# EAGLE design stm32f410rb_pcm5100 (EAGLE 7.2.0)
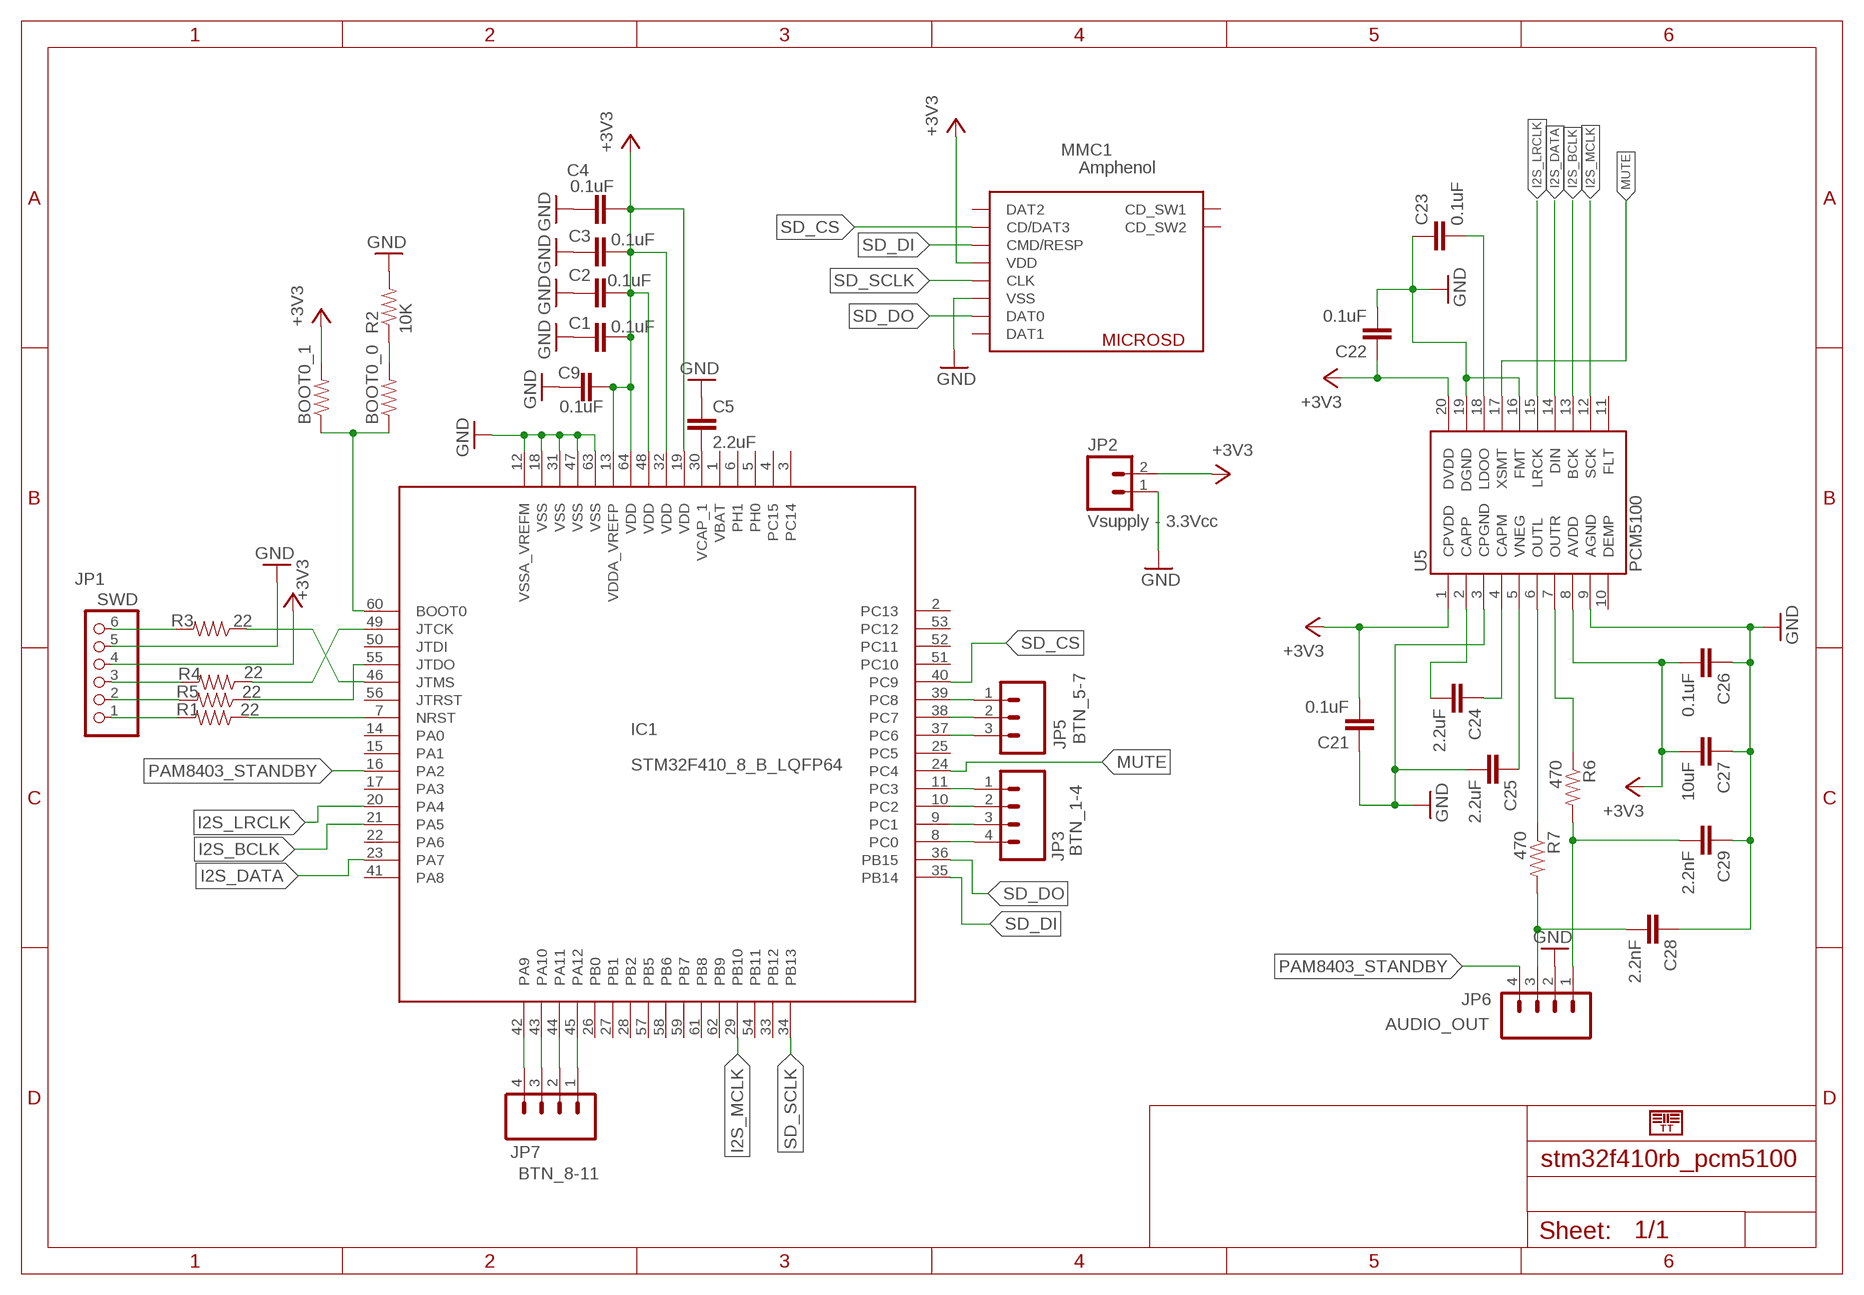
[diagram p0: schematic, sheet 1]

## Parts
BOOT0_0  RESISTOR0603-RES  [0603-RES]
BOOT0_1  RESISTOR0603-RES  [0603-RES]
C1  0.1uF  CAP0805  [0805]
C2  0.1uF  CAP0805  [0805]
C3  0.1uF  CAP0805  [0805]
C4  0.1uF  CAP0805  [0805]
C5  2.2uF  CAP0805  [0805]
C9  0.1uF  CAP0805  [0805]
C21  0.1uF  CAP0805  [0805]
C22  0.1uF  CAP0805  [0805]
C23  0.1uF  CAP0805  [0805]
C24  2.2uF  CAP0805  [0805]
C25  2.2uF  CAP0805  [0805]
C26  0.1uF  CAP0805  [0805]
C27  10uF  CAP0805  [0805]
C28  2.2nF  CAP0805  [0805]
C29  2.2nF  CAP0805  [0805]
IC1  STM32F410_8_B_LQFP64  [LQFP64]
JP1  SWD  PINHD-1X6  [1X06]
JP2  Vsupply - 3.3Vcc  M023.5MM  [SCREWTERMINAL-3.5MM-2]
JP3  BTN_1-4  M04SCREW  [SCREWTERMINAL-3.5MM-4]
JP5  BTN_5-7  M03SCREW  [SCREWTERMINAL-3.5MM-3]
JP6  AUDIO_OUT  M04SCREW  [SCREWTERMINAL-3.5MM-4]
JP7  BTN_8-11  M04SCREW  [SCREWTERMINAL-3.5MM-4]
MMC1  Amphenol  MICROSD_AMPHENOL  [MICROSD_AMPHENOL]
R1  22  RESISTOR0805-RES  [0805]
R2  10K  RESISTOR0805-RES  [0805]
R3  22  RESISTOR0805-RES  [0805]
R4  22  RESISTOR0805-RES  [0805]
R5  22  RESISTOR0805-RES  [0805]
R6  470  RESISTOR0805-RES  [0805]
R7  470  RESISTOR0805-RES  [0805]
U5  PCM5100  [PW_R-PDSO-G20]

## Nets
GND: C1.2 C2.2 C3.2 C4.2 C5.1 C9.2 C21.1 C22.2 C23.1 C25.2 C26.1 C27.1 C28.1 C29.1 IC1.12(VSSA_VREFM) IC1.18(VSS) IC1.31(VSS) IC1.47(VSS) IC1.63(VSS) JP1.5 JP2.1 JP6.2 MMC1.VSS R2.2 U5.3(CPGND) U5.9(AGND) U5.16(FMT) U5.19(DGND)
I2S_BCLK: IC1.21(PA5) U5.13(BCK)
I2S_DATA: IC1.23(PA7) U5.14(DIN)
I2S_LRCLK: IC1.20(PA4) U5.15(LRCK)
I2S_MCLK: IC1.29(PB10) U5.12(SCK)
LOUTL: C28.2 JP6.3 R7.2
LOUTR: C29.2 JP6.1 R6.2
MUTE: IC1.24(PC4) U5.17(XSMT)
N$1: IC1.11(PC3) JP3.1
N$2: IC1.10(PC2) JP3.2
N$3: IC1.9(PC1) JP3.3
N$4: IC1.8(PC0) JP3.4
N$5: C5.2 IC1.30(VCAP_1)
N$6: IC1.7(NRST) R1.1
N$7: IC1.49(JTCK) R4.1
N$8: IC1.55(JTDO) R5.1
N$9: IC1.46(JTMS) R3.1
N$10: BOOT0_0.2 R2.1
N$12: IC1.39(PC8) JP5.1
N$13: IC1.38(PC7) JP5.2
N$14: C23.2 U5.18(LDOO)
N$15: R6.1 U5.7(OUTR)
N$16: C24.2 U5.2(CAPP)
N$17: C24.1 U5.4(CAPM)
N$18: C25.1 U5.5(VNEG)
N$19: R7.1 U5.6(OUTL)
N$20: BOOT0_0.1 BOOT0_1.1 IC1.60(BOOT0)
N$21: IC1.37(PC6) JP5.3
N$22: IC1.45(PA12) JP7.1
N$23: IC1.44(PA11) JP7.2
N$24: IC1.43(PA10) JP7.3
N$25: IC1.42(PA9) JP7.4
N$26: JP1.6 R3.2
N$27: JP1.3 R4.2
N$28: JP1.2 R5.2
N$29: JP1.1 R1.2
PAM8403_STANDBY: IC1.16(PA2) JP6.4
SD_CS: IC1.40(PC9) MMC1.CD/DAT3
SD_DI: IC1.35(PB14) MMC1.CMD/RESP
SD_DO: IC1.36(PB15) MMC1.DAT0
SD_SCLK: IC1.34(PB13) MMC1.CLK
VCC: BOOT0_1.2 C1.1 C2.1 C3.1 C4.1 C9.1 C21.2 C22.1 C26.2 C27.2 IC1.13(VDDA_VREFP) IC1.19(VDD) IC1.32(VDD) IC1.48(VDD) IC1.64(VDD) JP1.4 JP2.2 MMC1.VDD U5.1(CPVDD) U5.8(AVDD) U5.20(DVDD) ; supply symbol labelled +3V3
Unconnected: IC1.1(VBAT) IC1.2(PC13) IC1.3(PC14) IC1.4(PC15) IC1.5(PH0) IC1.6(PH1) IC1.14(PA0) IC1.15(PA1) IC1.17(PA3) IC1.22(PA6) IC1.25(PC5) IC1.26(PB0) IC1.27(PB1) IC1.28(PB2) IC1.33(PB12) IC1.41(PA8) IC1.50(JTDI) IC1.51(PC10) IC1.52(PC11) IC1.53(PC12) IC1.54(PB11) IC1.56(JTRST) IC1.57(PB5) IC1.58(PB6) IC1.59(PB7) IC1.61(PB8) IC1.62(PB9) MMC1.CD_SW1 MMC1.CD_SW2 MMC1.DAT1 MMC1.DAT2 U5.10(DEMP) U5.11(FLT)

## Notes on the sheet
- TT

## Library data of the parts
BOOT0_0 BOOT0_1 R1-R7 = SparkFun-Passives:RESISTOR: Resistor
C1-C5 C9 C21-C29 = SparkFun-Passives:CAP: Capacitor
IC1 = pel_stm32:STM32F410_8_B_LQFP64: STM32F410_8_B_LQFP64.bsd edit this description Auto generated by make-symbol-device-package-bsdl.ulp Rev. 18 Source: STM32F410_8_B_LQFP64.bsd
JP1 = pinhead:PINHD-1X6: PIN HEADER
JP2 = SparkFun-Connectors:M02: Standard 2-pin 0.1" header. Use with; PROD_ID: CONN-08399
JP3 JP6 JP7 = SparkFun-Connectors:M04: Header 4 Standard 4-pin 0.1" header. Use with straight break away headers (SKU : PRT-00116), right angle break away headers (PRT-00553), swiss pins (PRT-00743), machine pins (PRT-00117), and female headers (PRT-00115). Molex polarized connector foot print use with SKU : PRT-08231 with associated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
JP5 = SparkFun-Connectors:M03: Header 3 Standard 3-pin 0.1" header. Use with straight break away headers (SKU : PRT-00116), right angle break away headers (PRT-00553), swiss pins (PRT-00743), machine pins (PRT-00117), and female headers (PRT-00115). Molex polarized connector foot print use with SKU : PRT-08232 with associated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
MMC1 = microsd_amphenol:MICROSD_AMPHENOL: AMPHENOL COMMERCIAL PRODUCTS The 114-00841-68 is a top mount microSD Memory Card Connector with gold-plated contact and tin-plated solder tail. http://ro.farnell.com/amphenol-commercial-products/114-00841-68/memory-card-connector-microsd/dp/2293708?CMP=i-ddd7-00001003
U5 = robertsonics:PCM5100: PCM5100 Stereo DAC

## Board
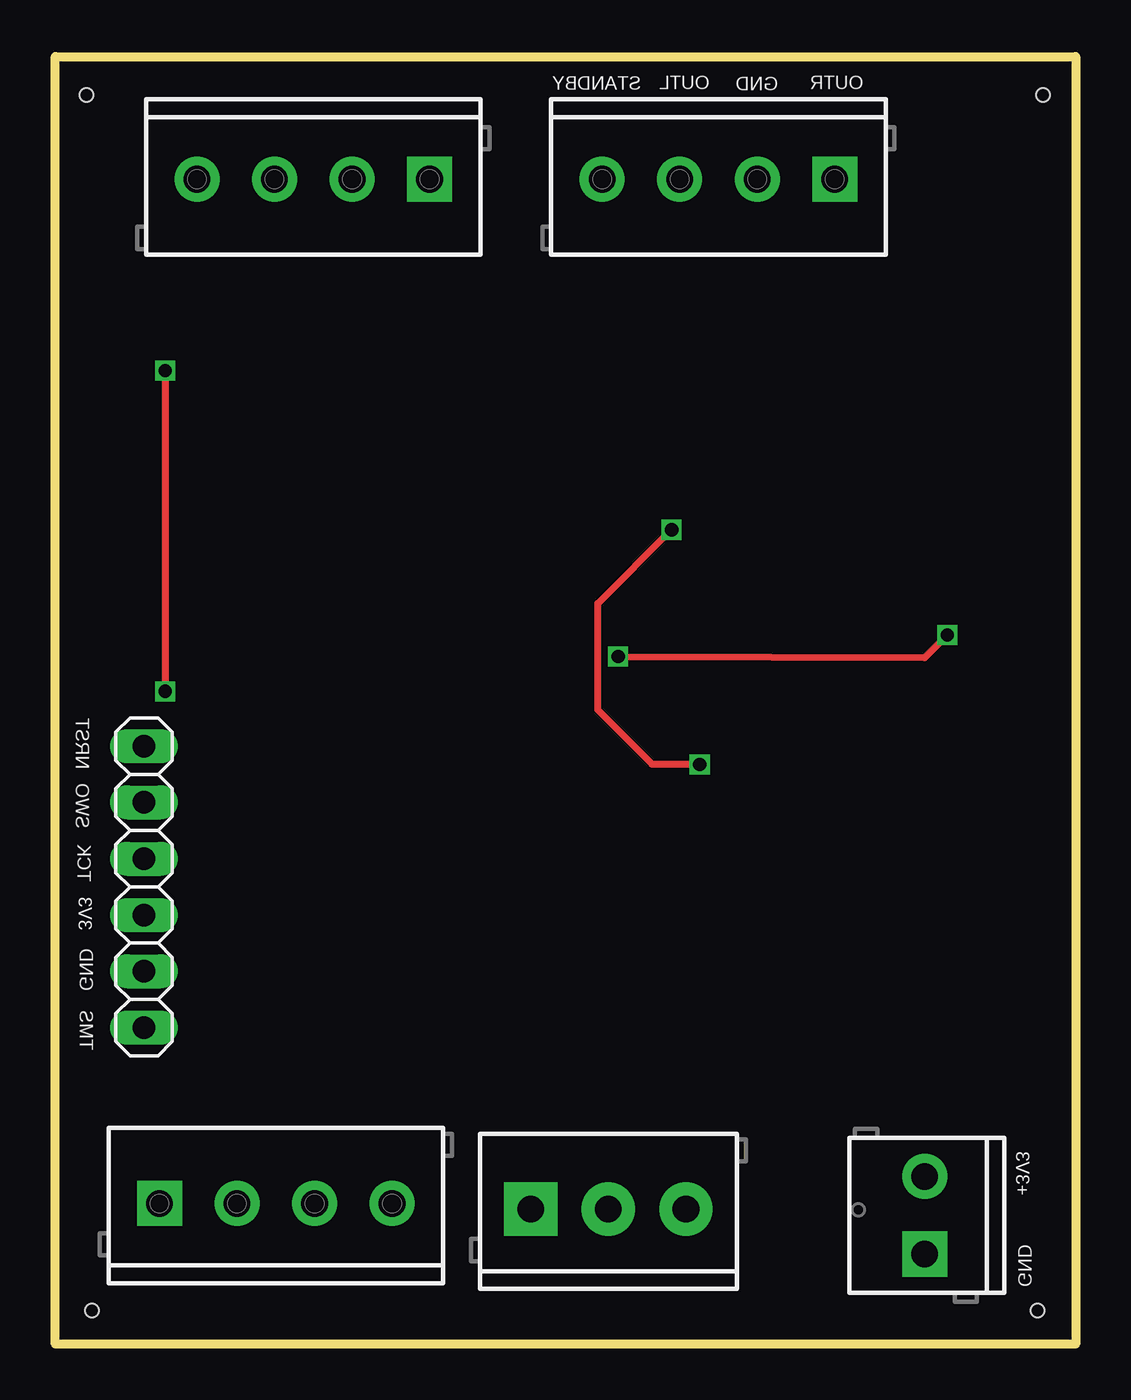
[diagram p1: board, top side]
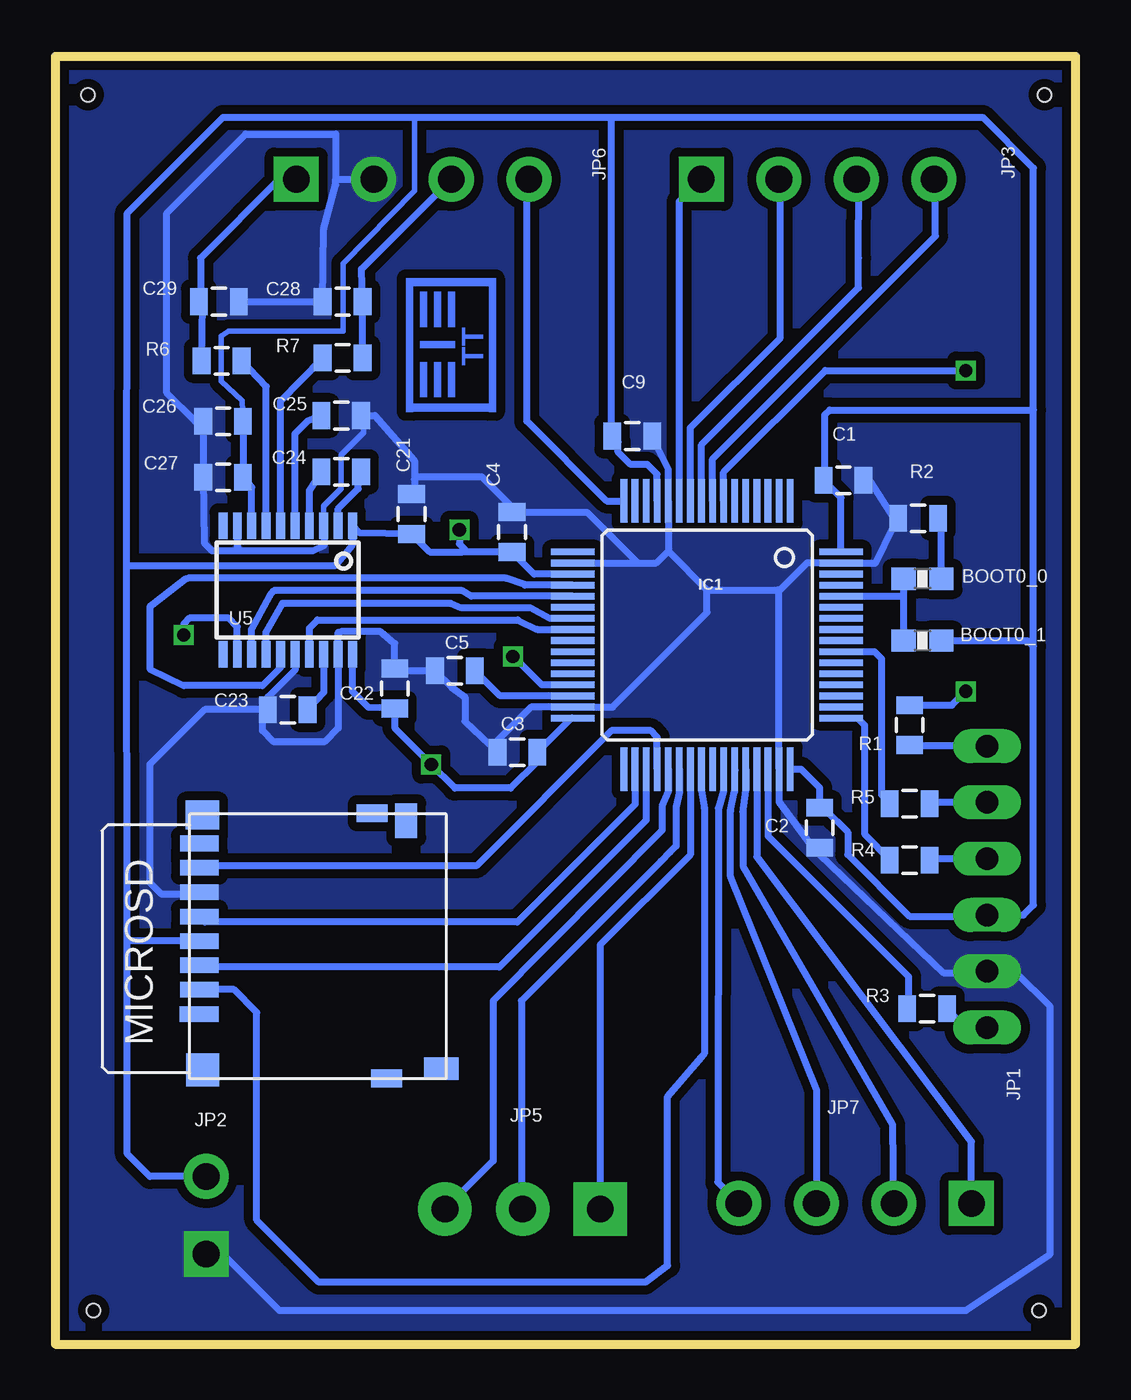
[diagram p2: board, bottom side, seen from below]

Size 46.05 x 58.17 mm. Coordinates in mm from the lower left corner, seen from the top.
Outline: 0,0 46.02,0 46.02,58.17 0,58.17
Outline: 0,58.09 0,0
Outline: 0,0 46.05,0 46.05,58.12 0,58.12 0,0
Copper layers (1*16): Top 0.035mm / dielectric 1.5mm / Bottom 0.035mm
Design rules "dirt_cheap_dirty_boards.v1 *": minimum track width 5mil, minimum drill 12mil, track to track 5mil, track to pad 5mil, pad to pad 5mil, via to via 5mil, smd to smd 0mil, copper to edge 10mil, drill to drill 10mil, minimum pad ring 10mil, minimum via ring 6mil, stop-mask expansion 2mil, vias tented up to drill 25mil, thermal gap 10mil
Holes 0.6 mm at 1.4,56.39 44.58,56.39 1.65,1.52 44.32,1.52

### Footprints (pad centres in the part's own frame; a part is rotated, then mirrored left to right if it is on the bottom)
0603-RES = smd 1.1 x 1: 1 -0.85,0; 2 0.85,0
0805 = smd 0.8 x 1.2: 1 -0.9,0; 2 0.9,0
LQFP64 = smd 1.962 x 0.3: 1 -6.05,3.75; 2 -6.05,3.25; 3 -6.05,2.75; 4 -6.05,2.25; 5 -6.05,1.75; 6 -6.05,1.25; 7 -6.05,0.75; 8 -6.05,0.25; 9 -6.05,-0.25; 10 -6.05,-0.75; 11 -6.05,-1.25; 12 -6.05,-1.75; 13 -6.05,-2.25; 14 -6.05,-2.75; 15 -6.05,-3.25; 16 -6.05,-3.75; 33 6.05,-3.75; 34 6.05,-3.25; 35 6.05,-2.75; 36 6.05,-2.25; 37 6.05,-1.75; 38 6.05,-1.25; 39 6.05,-0.75; 40 6.05,-0.25; 41 6.05,0.25; 42 6.05,0.75; 43 6.05,1.25; 44 6.05,1.75; 45 6.05,2.25; 46 6.05,2.75; 47 6.05,3.25; 48 6.05,3.75 | smd 0.3 x 1.962: 17 -3.75,-6.05; 18 -3.25,-6.05; 19 -2.75,-6.05; 20 -2.25,-6.05; 21 -1.75,-6.05; 22 -1.25,-6.05; 23 -0.75,-6.05; 24 -0.25,-6.05; 25 0.25,-6.05; 26 0.75,-6.05; 27 1.25,-6.05; 28 1.75,-6.05; 29 2.25,-6.05; 30 2.75,-6.05; 31 3.25,-6.05; 32 3.75,-6.05; 49 3.75,6.05; 50 3.25,6.05; 51 2.75,6.05; 52 2.25,6.05; 53 1.75,6.05; 54 1.25,6.05; 55 0.75,6.05; 56 0.25,6.05; 57 -0.25,6.05; 58 -0.75,6.05; 59 -1.25,6.05; 60 -1.75,6.05; 61 -2.25,6.05; 62 -2.75,6.05; 63 -3.25,6.05; 64 -3.75,6.05
1X06 = drill 1.016 long: 1 -6.35,0; 2 -3.81,0; 3 -1.27,0; 4 1.27,0; 5 3.81,0; 6 6.35,0
SCREWTERMINAL-3.5MM-2 = drill 1.2 pad 2.032 square: 1 0,0 | drill 1.2 pad 2.032: 2 3.5,0
SCREWTERMINAL-3.5MM-4 = drill 1.2 pad 2.032 square: 1 0,0 | drill 1.2 pad 2.032: 2 3.5,0; 3 7,0; 4 10.5,0
SCREWTERMINAL-3.5MM-3 = drill 1.2 pad 2.413 square: 1 0,0 | drill 1.2 pad 2.413: 2 3.5,0; 3 7,0
MICROSD_AMPHENOL = smd 0.7 x 1.75: CD/DAT3 2.1,-5.51; CLK -1.2,-5.51; CMD/RESP 1,-5.51; DAT0 -3.4,-5.51; DAT1 -4.5,-5.51; DAT2 3.21,-5.52; VDD -0.1,-5.51; VSS -2.3,-5.51 | smd 1 x 1.55: CD_SW1 5.66,5.41 | smd 1.55 x 1: CD_SW2 -5.53,3.82 | smd 1.3 x 1.5: NC1 -5.78,-5.38 | smd 1.5 x 1.5: NC2 5.72,-5.37 | smd 0.8 x 1.4: NC3 -5.86,2.29; NC_4 6.1,2.93
PW_R-PDSO-G20 = smd 0.4 x 1.2: 1 -2.925,-2.9; 2 -2.275,-2.9; 3 -1.625,-2.9; 4 -0.975,-2.9; 5 -0.325,-2.9; 6 0.325,-2.9; 7 0.975,-2.9; 8 1.625,-2.9; 9 2.275,-2.9; 10 2.925,-2.9; 11 2.925,2.9; 12 2.275,2.9; 13 1.625,2.9; 14 0.975,2.9; 15 0.325,2.9; 16 -0.325,2.9; 17 -0.975,2.9; 18 -1.625,2.9; 19 -2.275,2.9; 20 -2.925,2.9

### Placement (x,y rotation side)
BOOT0_0  6.91,34.54 0 bottom
BOOT0_1  6.91,31.75 0 bottom
C1  10.48,38.99 0 bottom
C2  11.56,23.3 270 bottom
C3  25.2,26.72 180 bottom
C4  25.44,36.65 90 bottom
C5  28.02,30.39 0 bottom
C9  20.02,40.98 0 bottom
C21  29.97,37.47 270 bottom
C22  30.73,29.59 90 bottom
C23  35.56,28.64 0 bottom
C24  33.15,39.37 0 bottom
C25  33.15,41.91 0 bottom
C26  38.48,41.66 0 bottom
C27  38.48,39.12 0 bottom
C28  33.08,47.05 0 bottom
C29  38.67,47.05 180 bottom
IC1  16.64,32 270 bottom
JP1  4,20.64 270 top
JP2  39.24,4.06 90 top
JP3  16.89,52.58 180 top
JP5  21.46,6.1 0 top
JP6  35.18,52.58 180 top
JP7  4.7,6.35 0 top
MMC1  34.04,18.1 270 bottom
R1  7.49,27.94 270 bottom
R2  7.11,37.27 180 bottom
R3  6.71,15.14 0 bottom
R4  7.49,21.84 0 bottom
R5  7.49,24.38 0 bottom
R6  38.54,44.39 180 bottom
R7  33.08,44.51 0 bottom
U5  35.56,34.04 180 bottom

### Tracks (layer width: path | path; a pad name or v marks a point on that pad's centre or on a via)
GND
  Bottom 0.254: U5.3 33.93,37.82 33.15,38.61 33.15,40.13 32.13,41.15 32.13,41.49 C25.2
  Bottom 0.305: 13.39,33.98 IC1.47 13.39,25.55 13.39,24.46 11.86,22.4 C2.2 11.56,22.1 5.97,16.76 4.06,16.76 JP1.5 3.94,16.76 2.67,16.76 1.14,15.24 1.14,4.06 4.95,1.52 35.94,1.52 38.48,4.06 JP2.1 | 18.39,35.79 IC1.12 18.39,39.49 C9.2 | 18.39,35.79 16.64,34.04 | 16.64,34.04 13.44,34.04 13.39,33.98 | IC1.18 19.76,35.25 | 19.76,35.25 18.92,35.25 18.39,35.79 | 8,37.31 R2.2 | 8.23,37.31 8.23,36.88 9.02,35.25 IC1.63 12.12,35.25 13.39,33.98 | 8.23,37.31 8.05,37.27 R2.2 | C29.1 C28.1 33.93,50.32 33.4,52.32 33.4,52.58 | C25.2 31.62,41.91 29.85,39.88 29.85,39.04 | 29.85,39.04 29.85,38.44 C21.1 | U5.9 37.84,35.93 37.72,35.81 | 37.72,35.81 34.42,35.81 33.91,36.07 33.91,36.91 U5.3 | 37.72,35.81 38.99,35.81 39.33,36.16 C27.1 C26.1 39.75,41.66 41.02,42.93 41.02,51.05 37.46,54.61 33.4,54.61 33.4,52.58 | 33.4,52.58 JP6.2 | C23.1 39.31,28.64 41.78,26.16 41.78,20.83 41.27,20.32 39.62,20.32 MMC1.VSS | C22.2 30.73,31.62 31.37,32.16 33.15,32.16 33.28,32.12 U5.19 33.28,27.8 33.91,27.18 36.2,27.18 36.7,27.69 36.7,28.35 C23.1 | U5.16 35.23,30.42 36.45,29.21 36.45,28.68 C23.1 | 30.71,30.42 C22.2 | 16.64,34.04 16.64,33.02 20.9,28.75 IC1.31 24.59,28.75 26.09,27.25 26.09,26.73 C3.2 27.56,28.11 27.56,29.21 28.16,29.63 C5.1 30.63,30.39 C22.2 | C1.2 9.63,38.94 9.27,38.94 8.23,37.31 | 8.23,37.31 R2.2 | 29.85,39.04 29.74,39.14 26.8,39.14 25.44,37.78 C4.2 22.06,37.55 19.76,35.25
  pour Bottom (isolate 0.406, no thermals): -0.03,58.19 46.05,58.19 46.05,-0.08 -0.03,-0.08
I2S_BCLK
  Bottom 0.305: U5.13 37.21,31.16 37.21,32.26 36.37,33.78 36.19,34.01 27.69,34.01 27.28,33.75 IC1.21
I2S_DATA
  Bottom 0.305: U5.14 36.53,32.17 35.81,33.43 28.19,33.43 27.71,33.22 24.61,33.22 23.74,32.75 IC1.23
I2S_LRCLK
  Bottom 0.305: U5.15 35.88,30.54 36.7,29.72 40.26,29.72 41.78,30.48 41.78,33.27 40.17,34.53 40.07,34.57 25.73,34.57 24.88,34.28 24.86,34.25 IC1.20
I2S_MCLK  (via drill 0.6)
  Top 0.305: v25.4,31.04 39.24,30.99 v40.26,32
  Bottom 0.305: IC1.29 24.09,29.75 25.02,30.68 v25.4,31.04 | U5.12 37.84,32.37 38.23,32.77 40,32.77 40.26,32.51 v40.26,32
LOUTL
  Bottom 0.305: R7.2 C28.2 32.23,48.52 JP6.3
LOUTR
  Bottom 0.305: R6.2 39.39,46.93 C29.2 39.5,47.08 39.5,49.02 35.94,52.58 JP6.1
MUTE
  Bottom 0.305: IC1.24 22.39,32.26 24.31,32.26 25.15,32.66 25.17,32.69 34.21,32.69 34.59,32.32 U5.17
N$1
  Bottom 0.305: IC1.11 17.89,51.58 JP3.1
N$2
  Bottom 0.305: JP3.2 13.33,52.52 13.33,45.41 17.39,41.36 IC1.10
N$3
  Bottom 0.305: IC1.9 16.89,40.59 9.8,47.68 9.8,49.02 9.78,52.47 JP3.3
N$4
  Bottom 0.305: IC1.8 16.39,39.95 6.33,50.01 6.33,52.51 JP3.4
N$5
  Bottom 0.305: IC1.30 25.98,29.25 C5.2
N$6  (via drill 0.6)
  Top 0.305: v4.95,43.94 v4.95,29.46
  Bottom 0.305: IC1.7 15.89,39.36 11.3,43.94 v4.95,43.94 | R1.1 5.58,28.84 v4.95,29.46
N$7
  Bottom 0.305: IC1.49 9.84,28.25 9.52,27.94 9.52,23.03 R4.1
N$8
  Bottom 0.305: IC1.55 9.08,31.25 8.76,30.94 8.76,24.8 R5.1
N$9
  Bottom 0.305: IC1.46 13.89,22.93 7.54,16.59 7.54,15.2 R3.1
N$10
  Bottom 0.305: BOOT0_0.2 6.06,37.12 R2.1
N$12
  Bottom 0.305: JP5.1 21.46,18.01 17.39,22.09 IC1.39
N$13
  Bottom 0.305: JP5.2 25.02,6.15 25.02,15.49 18.72,21.79 18.3,22.21 18.03,22.48 18.03,24.23 17.89,24.91 IC1.38
N$14
  Bottom 0.305: U5.18 33.93,29.41 C23.2
N$15
  Bottom 0.305: U5.7 36.53,43.23 R6.1
N$16
  Bottom 0.305: U5.2 33.28,37.71 32.38,38.61 32.38,39.03 C24.2
N$17
  Bottom 0.305: U5.4 34.59,38.53 C24.1
N$18
  Bottom 0.305: U5.5 35.23,41.09 34.67,41.66 C25.1
N$19
  Bottom 0.305: U5.6 35.88,42.56 R7.1
N$20
  Bottom 0.305: IC1.60 7.78,33.75 7.76,33.73 | BOOT0_1.1 7.76,33.73 | 7.76,33.73 BOOT0_0.1
N$21
  Bottom 0.305: JP5.3 26.29,8.27 26.29,15.49 18.67,23.19 18.67,24.26 18.39,24.95 IC1.37
N$22
  Bottom 0.305: JP7.1 4.7,9.14 14.39,22.01 IC1.45
N$23
  Bottom 0.305: IC1.44 14.88,24.99 15.01,23.98 15.01,21.59 8.25,9.91 JP7.2
N$24
  Bottom 0.305: JP7.3 11.7,6.86 | 11.7,6.86 11.7,7 | IC1.43 15.39,25.8 15.39,24.94 15.57,24.05 15.57,21.11 11.71,11.51 11.71,6.86 11.7,6.86
N$25
  Bottom 0.305: 15.89,7.04 JP7.4 16.15,7.3 16.13,24.18 15.89,24.95 IC1.42
N$26
  Bottom 0.305: JP1.6 4.1,14.39 5.06,14.39 R3.2
N$27
  Bottom 0.305: JP1.3 6.58,21.91 R4.2
N$28
  Bottom 0.305: JP1.2 6.58,24.45 R5.2
N$29
  Bottom 0.305: JP1.1 7.39,26.99 R1.2
PAM8403_STANDBY
  Bottom 0.305: JP6.4 24.77,52.49 24.77,41.66 21.17,38.06 IC1.16
SD_CS
  Bottom 0.305: MMC1.CD/DAT3 37.99,16 36.96,14.97 36.96,5.59 34.16,2.79 19.43,2.79 18.42,3.56 18.42,11.18 16.89,12.96 16.76,13.11 16.76,24.18 16.89,24.96 IC1.40
SD_DI
  Bottom 0.305: IC1.35 19.39,23.64 26.01,17.02 39.47,17.02 MMC1.CMD/RESP
SD_DO
  Bottom 0.305: IC1.36 18.89,27.4 19.18,27.69 20.96,27.69 27.05,21.59 39.45,21.59 MMC1.DAT0
SD_SCLK
  Bottom 0.305: IC1.34 19.89,24.36 25.2,19.05 39.3,19.05 MMC1.CLK
VCC  (via drill 0.6)
  Top 0.305: v29.08,26.16 26.92,26.16 26.92,26.19 24.49,28.63 24.49,33.43 v27.81,36.75
  Bottom 0.254: C26.2 37.63,42.58 38.56,43.46 38.56,45.49 38.23,45.72 33.07,45.72 33.07,48.77 29.85,52.07 29.85,55.37
  Bottom 0.305: U5.8 37.18,38.67 C27.2 C26.2 | v29.08,26.16 30.73,27.81 C22.1 31.92,28.74 32.64,29.46 U5.20 | 28.83,25.91 v29.08,26.16 | 42.8,18.29 42.8,8.58 41.78,7.56 JP2.2 | 42.8,18.29 42.82,35.13 | 42.82,35.13 42.8,51.05 38.48,55.37 29.85,55.37 20.96,55.37 | 42.82,35.13 33.43,35.13 32.63,36.07 U5.1 32.31,36.62 C21.2 29.16,35.75 27.67,35.75 | 1.91,31.5 1.91,19.81 2.35,19.37 JP1.4 4.06,19.3 7.49,19.3 10.29,22.1 10.29,23.11 11.33,24.15 C2.1 11.56,25.12 12.39,25.95 IC1.48 | 1.91,31.5 1.91,42.16 | 1.91,42.16 1.91,53.09 4.19,55.37 20.96,55.37 | BOOT0_1.2 2.16,31.75 1.91,31.5 | 1.91,42.16 11.1,42.16 11.33,41.94 11.33,39.04 C1.1 10.59,38.2 IC1.64 | 20.96,55.37 20.96,40.62 C9.1 20.65,40.72 20.65,40.26 20.09,39.7 19.33,39.7 18.89,39.26 IC1.13 | MMC1.VDD 42.71,18.2 42.8,18.29 | IC1.19 24.44,34.75 C4.1 27.67,35.75 | IC1.32 22.76,28.25 C3.1 24.3,26.3 25.5,25.09 28.02,25.09 v29.08,26.16 | 27.67,35.75 27.56,35.87 27.81,36.12 v27.81,36.75
(copper drawn outside any net)
  shapes: Bottom area x11

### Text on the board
Bottom: TT
tPlace: STANDBY | OUTL | GND | OUTR | NRST | SWO | TCK | 3V3 | GND | TMS | +3V3 | GND

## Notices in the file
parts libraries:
SparkFun-Passives: Licensing: CC v3.0 Share-Alike You are welcome to use this library for commercial purposes.
SparkFun-Connectors: Licensing: Creative Commons ShareAlike 4.0 International - https://creativecommons.org/licenses/by-sa/4.0
